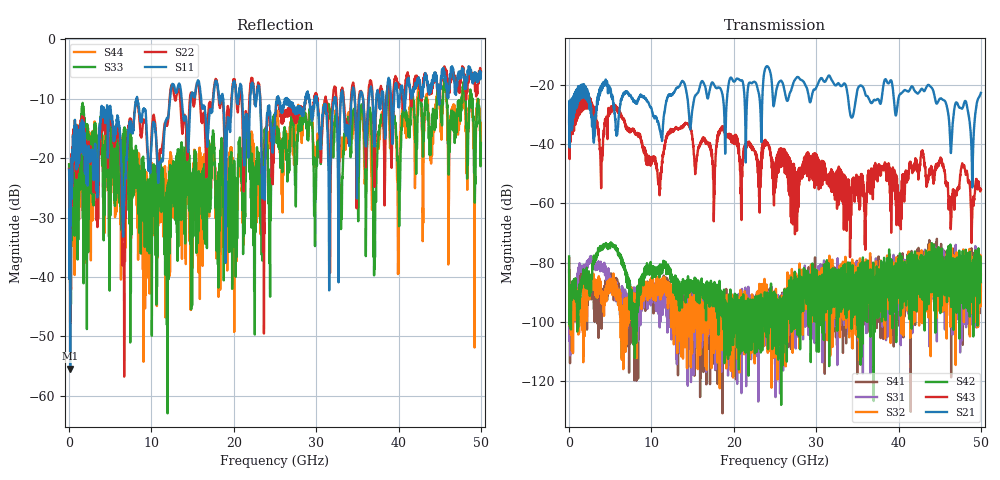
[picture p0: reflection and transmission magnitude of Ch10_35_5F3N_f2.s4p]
!Agilent Technologies,N5247A,US51170199,A.09.90.13
!Agilent N5247A: A.09.90.13
!Date: Wednesday, December 16, 2015 12:44:14
!Correction: S11(Full 4 Port(1,2,3,4))
!S12(Full 4 Port(1,2,3,4))
!S13(Full 4 Port(1,2,3,4))
!S14(Full 4 Port(1,2,3,4))
!S21(Full 4 Port(1,2,3,4))
!S22(Full 4 Port(1,2,3,4))
!S23(Full 4 Port(1,2,3,4))
!S24(Full 4 Port(1,2,3,4))
!S31(Full 4 Port(1,2,3,4))
!S32(Full 4 Port(1,2,3,4))
!S33(Full 4 Port(1,2,3,4))
!S34(Full 4 Port(1,2,3,4))
!S41(Full 4 Port(1,2,3,4))
!S42(Full 4 Port(1,2,3,4))
!S43(Full 4 Port(1,2,3,4))
!S44(Full 4 Port(1,2,3,4))
!S4P File: Measurements: <S11,S12,S13,S14>,
!<S21,S22,S23,S24>,
!<S31,S32,S33,S34>,
!<S41,S42,S43,S44>:
# Hz S  dB  R 50
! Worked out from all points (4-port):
!   3201 points, 10 MHz to 50 GHz, reference 50 ohm
!   strongest paths, dB at 10 MHz, 12.51 GHz, 25 GHz, 37.5 GHz, 50 GHz:
!     S21: -32.5, -23.4, -24.8, -24.9, -22.8
!     S43: -33.3, -35.1, -47.4, -47.5, -55.3
!     S42: -77.9, -85.0, -92.8, -86.0, -80.4
!     S32: -78.5, -101.9, -90.9, -82.7, -84.0
!     S31: -80.1, -95.8, -102.0, -86.0, -89.5
!     S41: -82.5, -91.8, -94.5, -92.7, -86.6
!   lowest |S11| = -55.5 dB at 135 MHz (marker M1), VSWR 1.00, Z = 50.1 + j0.16 ohm
!   |S11| at or under -10 dB: start of sweep to 8.23 GHz; 8.278 GHz to 12.26 GHz (3.981 GHz wide, 38.8 % of centre); 26.47 GHz to 28.7 GHz (2.237 GHz wide, 8.11 % of centre)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
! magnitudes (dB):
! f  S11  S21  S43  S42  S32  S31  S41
! 10 MHz  -22.0  -32.5  -33.3  -77.9  -78.5  -80.1  -82.5
! 135 MHz  -55.5  -32.7  -33.1  -98.8  -98.5  -111.3  -106.9
! 10.91 GHz  -22.7  -33.6  -54.1  -81.4  -88.5  -92.2  -95.9
! 14.19 GHz  -13.2  -21.7  -33.1  -87.0  -96.5  -95.9  -95.2
! 24.05 GHz  -12.5  -13.8  -39.5  -92.9  -102.4  -103.6  -91.8
! 48.94 GHz  -6.2  -52.0  -65.5  -80.4  -86.9  -84.2  -82.7
! 50 GHz  -5.6  -22.8  -55.3  -80.4  -84.0  -89.5  -86.6
